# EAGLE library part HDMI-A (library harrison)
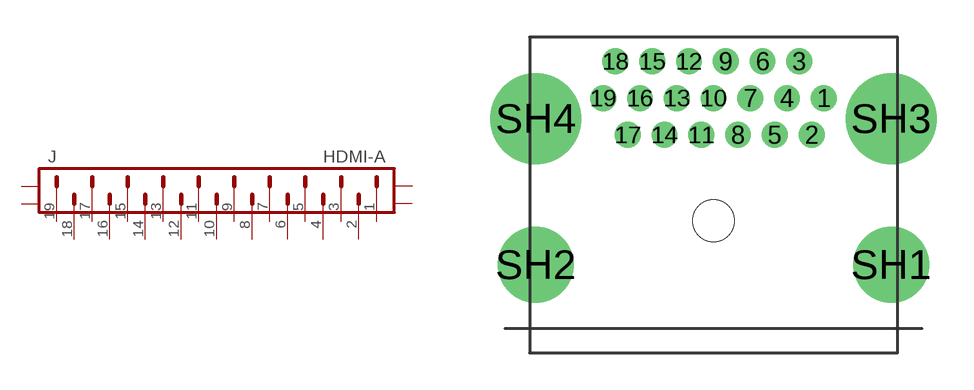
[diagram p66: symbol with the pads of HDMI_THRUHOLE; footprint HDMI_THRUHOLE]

Designator prefix J

## HDMI-A_THRU  [HDMI_THRUHOLE]
1  1  pas
2  2  pas
3  3  pas
4  4  pas
5  5  pas
6  6  pas
7  7  pas
8  8  pas
9  9  pas
10  10  pas
11  11  pas
12  12  pas
13  13  pas
14  14  pas
15  15  pas
16  16  pas
17  17  pas
18  18  pas
19  19  pas
SH1  SH1  pas
SH2  SH2  pas
SH3  SH3  pas
SH4  SH4  pas

## Footprint HDMI_THRUHOLE (pad centres in mm)
drill 0.55 pad 0.965: 1 4.5,5; 2 4,3.5; 3 3.5,6.5; 4 3,5; 5 2.5,3.5; 6 2,6.5; 7 1.5,5; 8 1,3.5; 9 0.5,6.5; 10 0,5; 11 -0.5,3.5; 12 -1,6.5; 13 -1.5,5; 14 -2,3.5; 15 -2.5,6.5; 16 -3,5; 17 -3.5,3.5; 18 -4,6.5; 19 -4.5,5
drill 2.1: SH1 7.25,-1.8; SH2 -7.25,-1.8
drill 2.7: SH3 7.25,4.16; SH4 -7.25,4.16
hole 1.7 at 0,0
